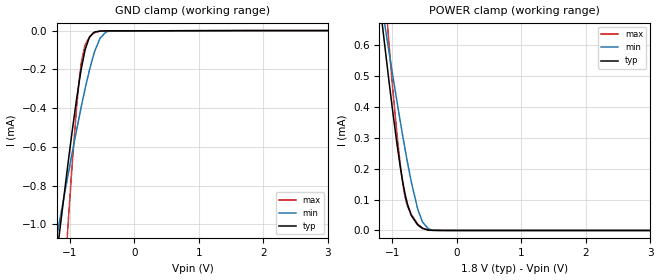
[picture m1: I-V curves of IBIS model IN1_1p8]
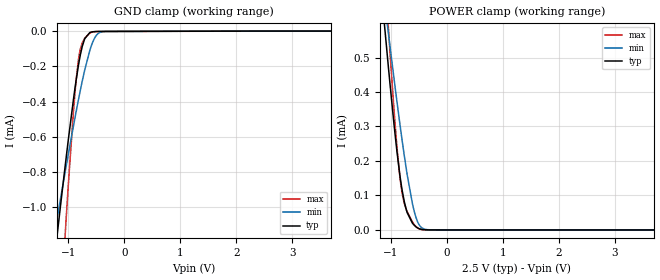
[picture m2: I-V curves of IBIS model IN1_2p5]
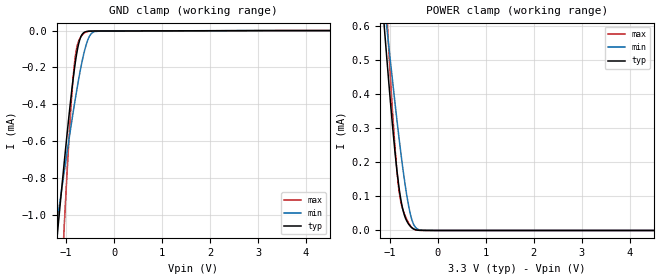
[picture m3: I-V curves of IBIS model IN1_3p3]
|Texas Instruments Incorporated
|ISO6721 General Purpose Dual-Channel Digital Isolator with Robust EMC
[IBIS Ver]   1.0
[File name]   iso6721.ibs
[Date]   21/03/2021
[File Rev]   2.0
[Source]
| Texas Instruments Incorporated.
| Analog-eLab Design Center, HPA
| 12500 TI Blvd
| Dallas, TX -75243
[Notes]   Revision History:
| Rev 1.0: 11/06/2020
| - Initial version of the model
| - Model generated from simulations in SPECTRE
| - Model names with a trailing _1p8 contain the model for 1.8V operation.
|   Model names with a trailing _2p5 contain the model for 2.5V operation.
|   Model names with a trailing _3p3 contain the model for 3.3V operation.
|   Model names with a trailing _5p0 contain the model for 5.0V operation.
[Notes]   Revision History:
| Rev 2.0: 21/03/2021
| - Updated for DWV package.
[Disclaimer]
| This model is designed as an aid for customers of Texas Instruments.
| TI and its licensors and suppliers make no warranties, either expressed
| or implied, with respect to this  model, including the warranties of
| merchantability or fitness for a particular purpose. The model is
| provided solely on an "as is" basis. The entire risk as to its quality
| and performance is with the customer.
| This model is subject to change without notice. Texas Instruments
| Incorporated is not responsible for updating this model.
[Copyright]
(C) Copyright 2020 Texas Instruments Incorporated.All rights reserved.
|  Component ISO6721DWV 8-Pin SOIC -DWV package
|  Part # ISO6721DWV
[Component]   IS06721DWV
[Manufacturer]   TI
[Package]   |8 SOIC - DWV package
|   typ   min   max
R_pkg   0.29774   0.1605   0.43022
L_pkg   4.3564E-09   3.8786E-09   4.7833E-09
C_pkg   6.85578E-13   3.7447E-13   1.4026E-12
[Pin]   signal_name   model_name   R_pin   L_pin   C_pin
1   VCC1   POWER   173.13m 4.2001n 0.58836p
2   OUTA   OUT   426.94m 4.7753n 0.4071p
3   INB   IN1   430.22m 4.7833n 0.42645p
4   GND1   GND   250.08m 4.5992n 1.4026p
5   GND2   GND   231.29m 4.228n  1.331p
6   OUTB   OUT   356.74m 4.1895n 0.39605p
7   INA   IN1   353.02m 4.1972n 0.37447p
8   VCC2   POWER   160.5m  3.8786n 0.55859p
|  Component ISO6721BD 8-Pin SOIC -D package
|  Part # ISO6721BD
[Component]   IS06721BD
[Manufacturer]   TI
[Package]   |8 SOIC - D package
|   typ   min   max
R_pkg   0.0649   0.0370   0.0830
L_pkg   1.9947n   1.8303n   2.2260n
C_pkg   0.3965p   0.3745p   0.4289p
[Pin]  signal_name   model_name   R_pin   L_pin   C_pin
1   VCC1   POWER   0.03706  1.83239n  0.42768p
2   OUTA   OUT   0.07937  1.93924n  0.37453p
3   INB   IN1   0.08295  1.99423n  0.37759p
4   GND1   GND   0.06024  2.20170n  0.40515p
5   GND2   GND   0.06024  2.22600n  0.40576p
6   OUTB   OUT   0.08295  1.99420n  0.37782p
7   INA   IN1   0.07937  1.93924n  0.37472p
8   VCC2   POWER   0.03703  1.83026n  0.42888p
|  Component ISO6721FDWV 8-Pin SOIC -DWV package
|  Part # ISO6721FDWV
[Component]   IS06721FDWV
[Manufacturer]   TI
[Package]   |8 SOIC - DWV package
|   typ   min   max
R_pkg   0.29774   0.1605   0.43022
L_pkg   4.3564E-09   3.8786E-09   4.7833E-09
C_pkg   6.85578E-13   3.7447E-13   1.4026E-12
[Pin]   signal_name   model_name   R_pin   L_pin   C_pin
1   VCC1   POWER   173.13m 4.2001n 0.58836p
2   OUTA   OUT   426.94m 4.7753n 0.4071p
3   INB   IN2   430.22m 4.7833n 0.42645p
4   GND1   GND   250.08m 4.5992n 1.4026p
5   GND2   GND   231.29m 4.228n  1.331p
6   OUTB   OUT   356.74m 4.1895n 0.39605p
7   INA   IN2   353.02m 4.1972n 0.37447p
8   VCC2   POWER   160.5m  3.8786n 0.55859p
|  Component ISO6721FBD 8-Pin SOIC -D package
|  Part # ISO6721FBD
[Component]   IS06721FBD
[Manufacturer]   TI
[Package]   |8 SOIC - D package
|   typ   min   max
R_pkg   0.0649   0.0370   0.0830
L_pkg   1.9947n   1.8303n   2.2260n
C_pkg   0.3965p   0.3745p   0.4289p
[Pin]  signal_name   model_name   R_pin   L_pin   C_pin
1   VCC1   POWER   0.03706  1.83239n  0.42768p
2   OUTA   OUT   0.07937  1.93924n  0.37453p
3   INB   IN2   0.08295  1.99423n  0.37759p
4   GND1   GND   0.06024  2.20170n  0.40515p
5   GND2   GND   0.06024  2.22600n  0.40576p
6   OUTB   OUT   0.08295  1.99420n  0.37782p
7   INA   IN2   0.07937  1.93924n  0.37472p
8   VCC2   POWER   0.03703  1.83026n  0.42888p|
[Model Selector] IN1
IN1_1p8   1.8V   digital Input
IN1_2p5   2.5V   digital Input
IN1_3p3   3.3V   digital Input
IN1_5p0   5.0V   digital Input
[Model Selector] IN2
IN2_1p8   1.8V   digital Input
IN2_2p5   2.5V   digital Input
IN2_3p3   3.3V   digital Input
IN2_5p0   5.0V   digital Input
[Model Selector] OUT
OUT_1p8   1.8V   digital Output
OUT_2p5   2.5V   digital Output
OUT_3p3   3.3V   digital Output
OUT_5p0   5.0V   digital Output
| Models and submodels in the file (12): IN1_1p8 (Input), IN1_2p5 (Input), IN1_3p3 (Input), IN1_5p0 (Input), IN2_1p8 (Input), IN2_2p5 (Input), IN2_3p3 (Input), IN2_5p0 (Input), OUT_1p8 (3-state), OUT_2p5 (3-state), OUT_3p3 (3-state), OUT_5p0 (3-state)
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[Model]   IN1_1p8
Model_type   Input
Vinl = 0.54
Vinh = 1.26
|   typ   min   max
C_comp   0.00095pF   0.00076pF   0.0142pF
|  Where Nom  PVT is Nominal Process, 1.8V,  27C
|   Fast PVT is Strong Process,  1.89,  -40C
|   Slow PVT is Weak Process,   1.71V, 150C
[Model spec]
|subparameter
Vinl   0.54   0.513   0.567
Vinh   1.26   1.197   1.323
[Voltage Range]   1.8   1.71   1.89
|Junction Temperature
[Temperature Range]   27   150   -40
[Power Clamp Reference]   1.8   1.71   1.89
[GND Clamp Reference]   0   0   0
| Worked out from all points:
|   GND clamp passes 1 mA (typ) near -1.14 V on its own axis
|   POWER clamp passes 1 mA (typ) near -1.34 V on its own axis
[GND Clamp]
|   Voltage   I(typ)   I(min)   I(max)
-1.8V     -2.874mA   -2.195mA   -5.336mA
-1.184V   -1.11mA    -1.03mA    -1.821mA
-1.163V   -1.051mA   -990.6uA   -1.705mA
-1.028V   -686uA     -745.6uA   -1.004mA
-898.2mV  -361.3uA   -518.9uA   -411.1uA
-828mV    -209.5uA   -402uA     -181.4uA
-757.8mV  -93.79uA   -292.1uA   -71.12uA
-698.4mV  -36.2uA    -207.5uA   -35.59uA
-633.6mV  -10.97uA   -127.9uA   -14.52uA
-531mV    -2.469uA   -39.62uA   -2.975uA
-369mV    -1.445uA   -2.669uA   -1.543uA
3.6V      0A         0A         0A
[POWER Clamp]
|   Voltage   I(typ)   I(min)   I(max)
-1.8V     1.872mA    1.618mA    2.869mA
-1.179V   709.8uA    751.5uA    957.6uA
-1.055V   490uA      584.3uA    612.9uA
-919.8mV  269uA      408.1uA    296.9uA
-871.2mV  199.5uA    346.9uA    204.2uA
-817.2mV  133.9uA    281.2uA    125.6uA
-768.6mV  88.65uA    224.9uA    81.75uA
-703.8mV  48uA       155.6uA    51.14uA
-612mV    19.26uA    74.45uA    22.69uA
-531mV    6.785uA    27.03uA    7.136uA
-293.4mV  209.8nA    425.9nA    202.8nA
3.6V      0A         0A         0A
|   IN1_2p5 Model
[Model]   IN1_2p5
Model_type   Input
Vinl = 0.75
Vinh = 1.75
|   typ   min   max
C_comp   0.00095pF   0.00076pF   0.015pF
|  Where Nom  PVT is Nominal Process, 2.5V,   27C
|   Fast PVT is Strong Process,  2.25,   -340C
|   Slow PVT is Weak Process,   2.75V,  150C
[Model spec]
|subparameter
Vinl   0.75   0.675   0.825
Vinh   1.75   1.575   1.925
[Voltage Range]   2.5   2.25   2.75
|Junction Temperature
[Temperature Range]   27   150   -40
[Power Clamp Reference]   2.5   2.25   2.75
[GND Clamp Reference]   0   0   0
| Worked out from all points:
|   GND clamp passes 1 mA (typ) near -1.14 V on its own axis
[GND Clamp]
|   Voltage   I(typ)   I(min)   I(max)
-2.5V     -4.931mA   -3.55mA    -9.461mA
-1.232V   -1.244mA   -1.119mA   -2.084mA
-1.12V    -933.5uA   -912.3uA   -1.477mA
-1.038V   -711.7uA   -763uA     -1.052mA
-910mV    -389.1uA   -539.1uA   -459uA
-820mV    -194.3uA   -389.1uA   -163uA
-782.5mV  -129.3uA   -329.8uA   -97.62uA
-707.5mV  -42.82uA   -219.9uA   -40.05uA
-617.5mV  -8.649uA   -110.7uA   -11.7uA
-497.5mV  -2.387uA   -23.45uA   -2.737uA
-355mV    -1.896uA   -2.716uA   -2.116uA
5V        0A         0A         0A
[POWER Clamp]
|   Voltage   I(typ)   I(min)   I(max)
-2.5V     3.216mA    2.616mA    5.089mA
-1.113V   590.9uA    661.5uA    768.3uA
-1.067V   512uA      601.2uA    646.2uA
-1.03V    447.5uA    551.4uA    549.6uA
-902.5mV  243.4uA    386.1uA    262.1uA
-842.5mV  162.8uA    311.7uA    158.7uA
-805mV    121.3uA    266.8uA    112.2uA
-722.5mV  57.6uA     174.8uA    58.38uA
-617.5mV  20.43uA    78.61uA    24.1uA
-497.5mV  3.903uA    15.71uA    3.749uA
-257.5mV  171.2nA    276.9nA    172.3nA
5V        0A         0A         0A
|   IN1_3p3 Model
[Model]   IN1_3p3
Model_type   Input
Vinl = 0.99
Vinh = 2.31
|   typ   min   max
C_comp   0.00096pF   0.00076pF   0.016pF
|  Where Nom  PVT is Nominal Process, 3.3V,   27C
|   Fast PVT is Strong Process,  3.6,   -40C
|   Slow PVT is Weak Process,   3.0V,   150C
[Model spec]
|subparameter
Vinl   0.99   0.9   1.08
Vinh   2.31   2.1   2.52
[Voltage Range]   3.3   3   3.6
|Junction Temperature
[Temperature Range]   27   150   -40
[Power Clamp Reference]   3.3   3   3.6
[GND Clamp Reference]   0   0   0
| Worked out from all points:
|   GND clamp passes 1 mA (typ) near -1.14 V on its own axis
|   POWER clamp passes 1 mA (typ) near -1.34 V on its own axis
[GND Clamp]
|   Voltage   I(typ)   I(min)   I(max)
-3.3V     -7.303mA   -5.115mA   -14.21mA
-1.211V   -1.185mA   -1.08mA    -1.967mA
-1.152V   -1.02mA    -970.3uA   -1.646mA
-1.112V   -912uA     -897.9uA   -1.436mA
-1.033V   -699.6uA   -754.9uA   -1.03mA
-904.2mV  -375.5uA   -529.2uA   -435.5uA
-815.1mV  -185.3uA   -381.3uA   -152.7uA
-716.1mV  -49.91uA   -231.9uA   -44.58uA
-597.3mV  -6.774uA   -90.92uA   -9.051uA
-458.7mV  -2.634uA   -12.21uA   -2.924uA
-260.7mV  -2.357uA   -2.487uA   -2.627uA
6.6V      0A         0A         0A
[POWER Clamp]
|   Voltage   I(typ)   I(min)   I(max)
-3.3V     4.765mA    3.768mA    7.646mA
-1.132V   625.4uA    687.7uA    822.6uA
-1.102V   572.7uA    647.7uA    739.9uA
-1.082V   538uA      621.1uA    686uA
-1.023V   435.6uA    542.1uA    532.2uA
-894.3mV  231.5uA    375.8uA    246.2uA
-805.2mV  121.5uA    267uA      112.4uA
-716.1mV  54.13uA    168.1uA    55.82uA
-617.1mV  20.34uA    78.3uA     23.99uA
-547.8mV  8.703uA    34.54uA    9.499uA
-468.6mV  2.306uA    9.387uA    2.038uA
6.6V      0A         0A         0A
